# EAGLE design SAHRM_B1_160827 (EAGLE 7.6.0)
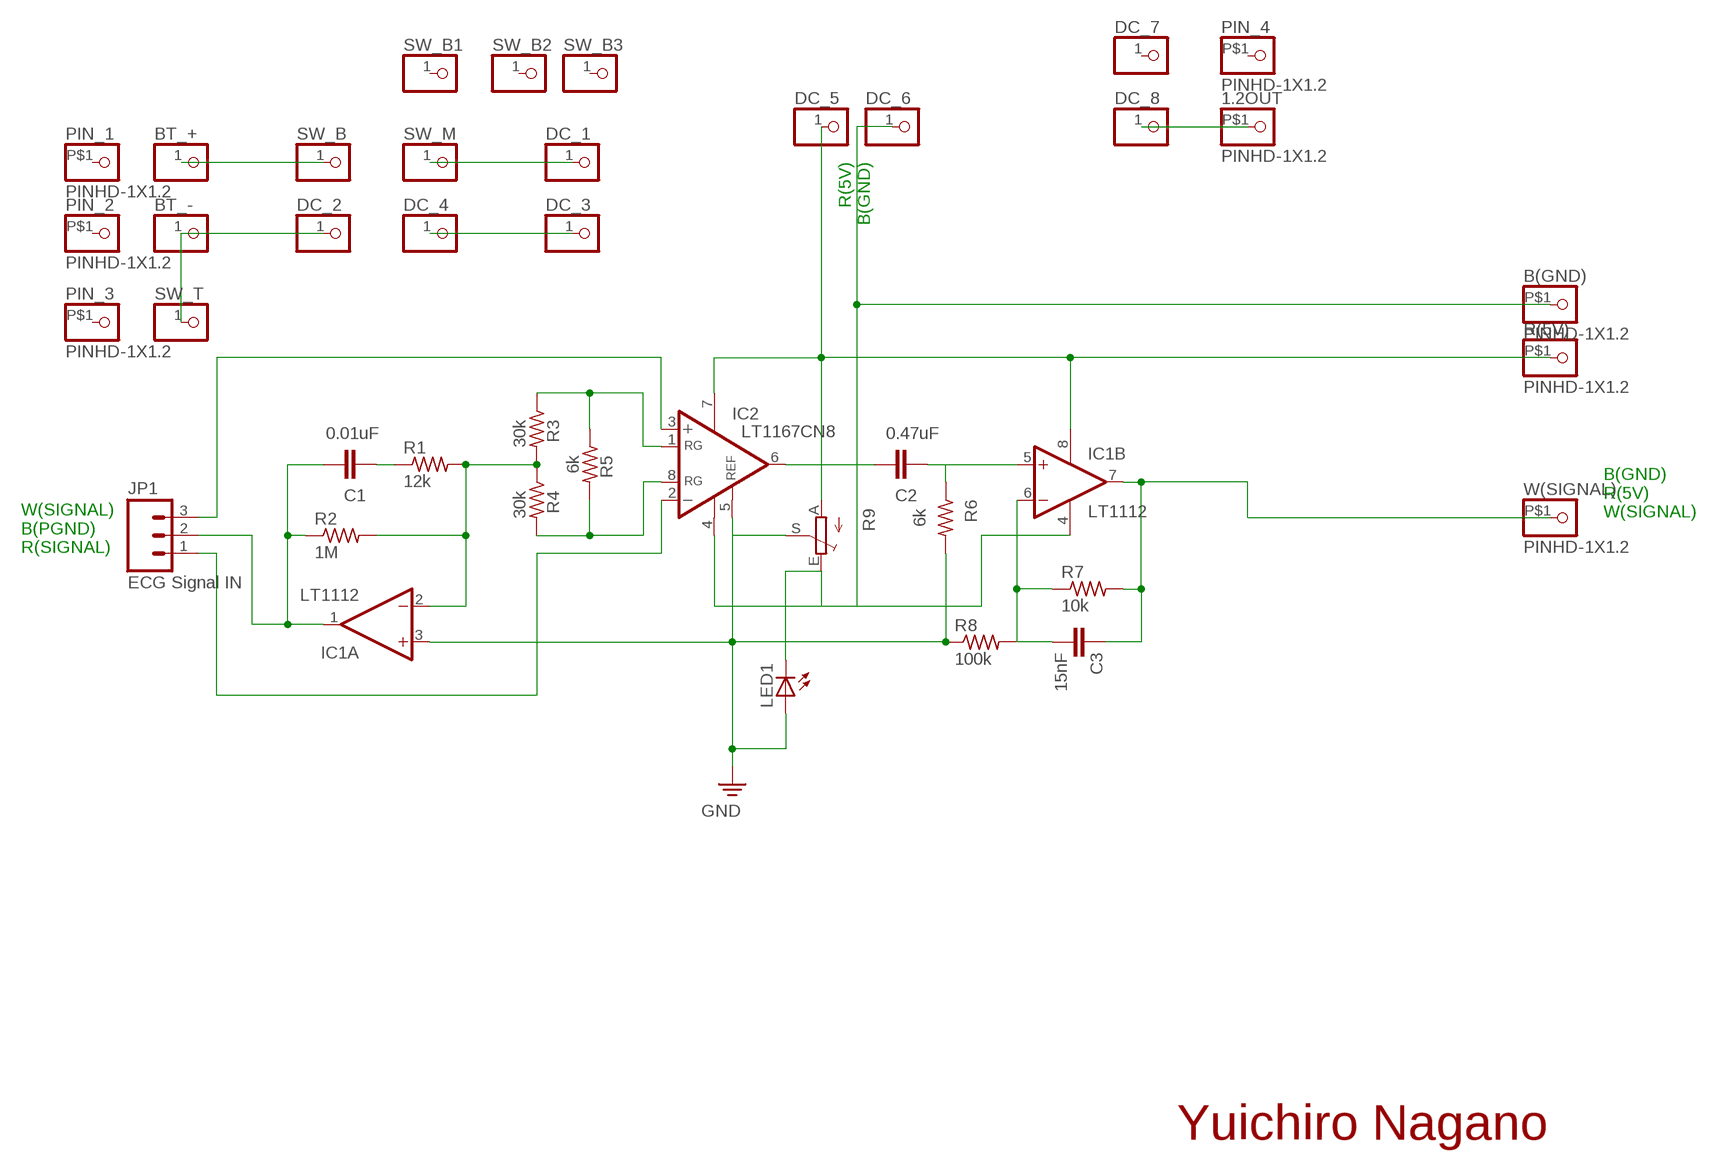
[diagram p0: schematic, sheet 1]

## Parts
1.2OUT  PINHD-1X1.2  [1X01.2]
B(GND)  PINHD-1X1.2  [1X01.2]
BT_+  PINHD-1X1  [1X01]
BT_-  PINHD-1X1  [1X01]
C1  0.01uF  C2,5-3  [C2.5-3]
C2  0.47uF  C2,5-3  [C2.5-3]
C3  15nF  C2,5-3  [C2.5-3]
DC_1  PINHD-1X1  [1X01]
DC_2  PINHD-1X1  [1X01]
DC_3  PINHD-1X1  [1X01]
DC_4  PINHD-1X1  [1X01]
DC_5  PINHD-1X1  [1X01]
DC_6  PINHD-1X1  [1X01]
DC_7  PINHD-1X1  [1X01]
DC_8  PINHD-1X1  [1X01]
IC1  LT1112  2AMP_P8+4N  [DIL08]
IC2  LT1167CN8  LT1168CN8  [DIL08]
JP1  ECG Signal IN  M03PTH  [1X03]
LED1  LED3MM  [LED3MM]
PIN_1  PINHD-1X1.2  [1X01.2]
PIN_2  PINHD-1X1.2  [1X01.2]
PIN_3  PINHD-1X1.2  [1X01.2]
PIN_4  PINHD-1X1.2  [1X01.2]
R1  12k  R-US_0204/2V  [0204V]
R2  1M  R-US_0204/2V  [0204V]
R3  30k  R-US_0204/2V  [0204V]
R4  30k  R-US_0204/2V  [0204V]
R5  6k  R-US_0204/2V  [0204V]
R6  6k  R-US_0204/2V  [0204V]
R7  10k  R-US_0204/2V  [0204V]
R8  100k  R-US_0204/2V  [0204V]
R9  TRIM_EU-B25P  [B25P]
R(5V)  PINHD-1X1.2  [1X01.2]
SW_B  PINHD-1X1  [1X01]
SW_B1  PINHD-1X1  [1X01]
SW_B2  PINHD-1X1  [1X01]
SW_B3  PINHD-1X1  [1X01]
SW_M  PINHD-1X1  [1X01]
SW_T  PINHD-1X1  [1X01]
W(SIGNAL)  PINHD-1X1.2  [1X01.2]

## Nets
B1: IC1.3(A:+IN) IC2.5(REF) LED1.A R6.2 R8.1 R9.S ; supply symbol labelled GND
N$1: C1.2 IC1.1(A:OUT) JP1.2 R2.1
N$2: IC2.3(+IN) JP1.3
N$3: IC1.2(A:-IN) R1.2 R2.2 R3.2 R4.1
N$4: IC2.1(RG) R3.1 R5.1
N$5: IC2.8(RG) R4.2 R5.2
N$6: IC2.2(-IN) JP1.1
N$7: 1.2OUT.P$1(1.1) DC_8.1
N$8: C2.2 IC2.6(OUT)
N$9: C2.1 IC1.5(B:+IN) R6.1
N$10: C3.2 IC1.6(B:-IN) R7.1 R8.2
N$11: C1.1 R1.1
N$15: DC_5.1 IC1.8(P:V+) IC2.7(V+) R9.A R(5V).P$1(1.1)
N$16: C3.1 IC1.7(B:OUT) R7.2 W(SIGNAL).P$1(1.1)
N$17: B(GND).P$1(1.1) DC_6.1 IC1.4(P:V-) IC2.4(V-) LED1.K(C) R9.E
N$27: BT_+.1 SW_B.1
N$28: BT_-.1 DC_2.1 SW_T.1
N$34: DC_1.1 SW_M.1
N$37: DC_3.1 DC_4.1
Unconnected: DC_7.1 PIN_1.P$1(1.1) PIN_2.P$1(1.1) PIN_3.P$1(1.1) PIN_4.P$1(1.1) SW_B1.1 SW_B2.1 SW_B3.1

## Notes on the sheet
- R(5V)
  B(GND)
- B(GND)
  R(5V)
  W(SIGNAL)
- W(SIGNAL)
  B(PGND)
  R(SIGNAL)
- Yuichiro Nagano

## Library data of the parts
1.2OUT B(GND) PIN_1-PIN_4 R(5V) W(SIGNAL) = pinhead:PINHD-1X1.2
BT_+ BT_- DC_1-DC_8 SW_B SW_B1-SW_B3 SW_M SW_T = adafruit:PINHD-1X1: Pin header 1x1 for 0.1" spacing
C1-C3 = capacitor-wima:C: CAPACITOR
IC1 = linear:2AMP_P8+4: OP AMP
IC2 = linear-technology:LT1168: Low Power, Single Resistor Gain Programmable, Precision Instrumentation Amplifier SourcE: LT1168.pdf; MPN: LT1168CN8#PBF; OC_FARNELL: 1330587; OC_NEWARK: 57M2327
JP1 = SparkFun-Connectors:M03: Header 3 Standard 3-pin 0.1" header. Use with straight break away headers (SKU : PRT-00116), right angle break away headers (PRT-00553), swiss pins (PRT-00743), machine pins (PRT-00117), and female headers (PRT-00115). Molex polarized connector foot print use with SKU : PRT-08232 with associated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
LED1 = adafruit:LED: LED
R1-R8 = resistor:R-US_: RESISTOR, American symbol
R9 = pot:TRIM_EU-: POTENTIOMETER

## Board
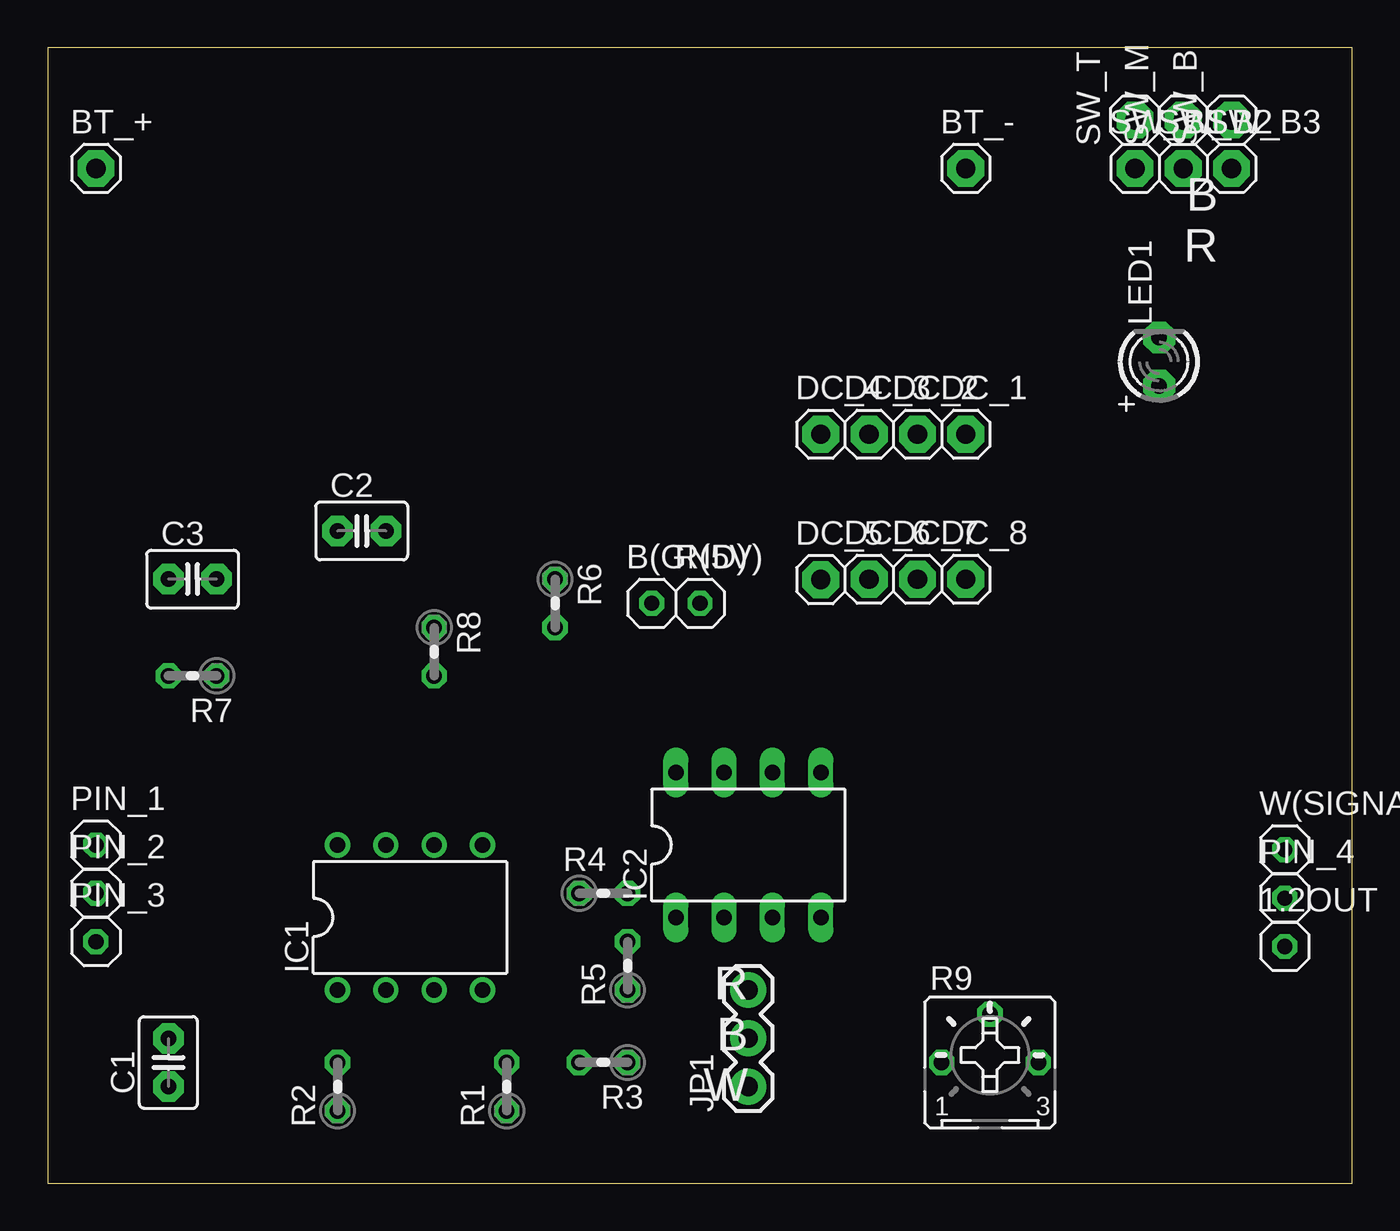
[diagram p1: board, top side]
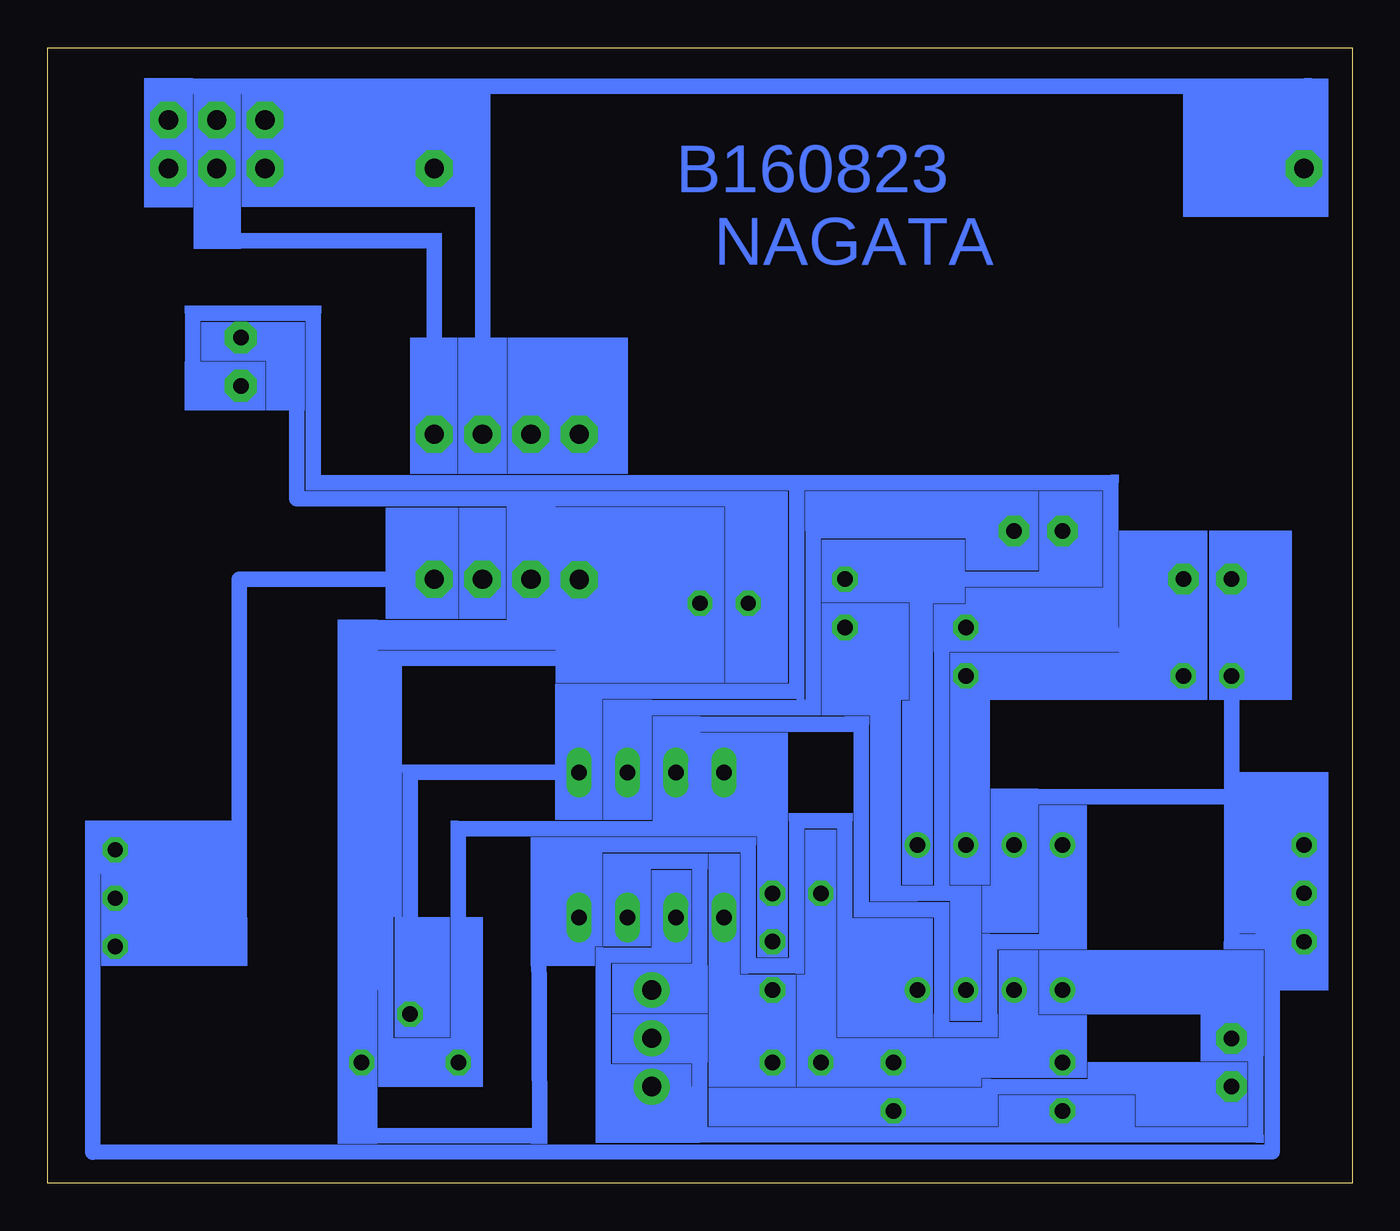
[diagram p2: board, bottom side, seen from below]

Size 68.58 x 59.69 mm. Coordinates in mm from the lower left corner, seen from the top.
Outline: 0,0 68.58,0 68.58,59.69 0,59.69 0,0
Copper layers (1*16): Top 0.035mm / dielectric 1.5mm / Bottom 0.035mm
Design rules "Fusion_eagle_rule_v1.1 *": minimum track width 32mil, minimum drill 12mil, track to track 6mil, track to pad 6mil, pad to pad 6mil, via to via 6mil, smd to smd 0mil, copper to edge 10mil, drill to drill 10mil, minimum pad ring 10mil, minimum via ring 6mil, stop-mask expansion 2mil, vias tented up to drill 100mil, thermal gap 10mil

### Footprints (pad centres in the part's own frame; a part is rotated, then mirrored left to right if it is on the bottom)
1X01.2 = drill 0.8 octagon: P$1 0,0
1X01 = drill 1.016 pad 1.93 octagon: 1 0,0
C2.5-3 = drill 0.813 pad 1.6 octagon: 1 -1.27,0; 2 1.27,0
DIL08 = drill 0.813 pad 1.27: 1 -3.81,-3.81; 2 -1.27,-3.81; 3 1.27,-3.81; 4 3.81,-3.81; 5 3.81,3.81; 6 1.27,3.81; 7 -1.27,3.81; 8 -3.81,3.81
DIL08' = drill 0.813 long: 1 -3.81,-3.81; 2 -1.27,-3.81; 3 1.27,-3.81; 4 3.81,-3.81; 5 3.81,3.81; 6 1.27,3.81; 7 -1.27,3.81; 8 -3.81,3.81
1X03 = drill 1.016 pad 1.88: 1 0,0; 2 2.54,0; 3 5.08,0
LED3MM = drill 0.813 pad 1.676 octagon: A -1.27,0; K 1.27,0
0204V = drill 0.813 octagon: 1 -1.27,0; 2 1.27,0
B25P = drill 0.813 octagon: A -2.54,0; E 2.54,0; S 0,2.54

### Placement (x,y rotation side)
1.2OUT  65.02,12.45 0 top
B(GND)  31.75,30.48 0 top
BT_+  2.54,53.34 0 top
BT_-  48.26,53.34 0 top
C1  6.35,6.35 90 top
C2  16.51,34.29 0 top
C3  7.62,31.75 0 top
DC_1  48.26,39.37 0 top
DC_2  45.72,39.37 0 top
DC_3  43.18,39.37 0 top
DC_4  40.64,39.37 0 top
DC_5  40.64,31.72 0 top
DC_6  43.18,31.75 0 top
DC_7  45.72,31.75 0 top
DC_8  48.26,31.75 0 top
IC1  19.05,13.97 0 top
IC2  LT1167CN8  [DIL08']  36.83,17.78 0 top
JP1  36.83,5.08 90 top
LED1  58.42,43.18 90 top
PIN_1  2.54,17.78 0 top
PIN_2  2.54,15.24 0 top
PIN_3  2.54,12.7 0 top
PIN_4  65.02,14.99 0 top
R1  24.13,5.08 90 top
R2  15.24,5.08 90 top
R3  29.21,6.35 180 top
R4  29.21,15.24 0 top
R5  30.48,11.43 90 top
R6  26.67,30.48 270 top
R7  7.62,26.67 180 top
R8  20.32,27.94 270 top
R9  49.53,6.35 0 top
R(5V)  34.29,30.48 0 top
SW_B  62.23,55.88 90 top
SW_B1  57.15,53.34 0 top
SW_B2  59.69,53.34 0 top
SW_B3  62.23,53.34 0 top
SW_M  59.69,55.88 90 top
SW_T  57.15,55.88 90 top
W(SIGNAL)  65.02,17.53 0 top

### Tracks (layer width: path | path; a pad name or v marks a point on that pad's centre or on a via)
B1
  Bottom 0.813: LED1.A 60.96,41.91 60.96,45.72 54.61,45.72 54.61,36.83 29.21,36.83 | 29.21,36.83 12.7,36.83 12.7,29.21 R8.1 21.59,29.21 21.59,15.24 | 29.21,36.83 29.21,25.86 40.64,25.86 IC2.5 49.53,21.59 R9.S | IC1.3 20.32,15.24 21.59,15.24 | R6.2 24.13,29.21 24.13,15.24 21.59,15.24
N$1
  Bottom 0.813: JP1.2 34.29,7.62 34.29,2.54 15.24,2.54 | 15.24,2.54 5.08,2.54 5.08,7.62 C1.2 6.35,10.16 IC1.1 | R2.1 15.24,2.54
N$2
  Bottom 0.813: IC2.3 38.1,16.92 34.29,16.92 34.29,10.16 JP1.3
N$3
  Bottom 0.813: 17.78,6.35 R1.2 R3.2 R4.1 | 17.78,6.35 R2.2 | 17.78,6.35 IC1.2
N$4
  Bottom 0.813: R3.1 R5.1 33.02,10.16 IC2.1
N$5
  Bottom 0.813: R5.2 R4.2 30.48,21.59 IC2.8
N$6
  Bottom 0.813: IC2.2 35.56,11.99 39.37,11.99 39.37,5.08 JP1.1
N$7
  Bottom 0.813: DC_8.1 58.5,31.75 58.5,12.42 65.02,12.42 1.2OUT.P$1
N$8
  Bottom 0.813: C2.2 28.35,34.29 28.35,24.99 38.1,24.99 IC2.6
N$9
  Bottom 0.813: C2.1 15.24,31.75 R6.1 22.86,31.75 IC1.5
N$10
  Bottom 0.813: C3.2 R7.1 R8.2 IC1.6
N$11
  Bottom 0.813: C1.1 19.05,5.08 19.05,3.81 R1.1
N$15
  Bottom 0.813: DC_5.1 40.64,30.48 | 40.64,30.48 40.64,27.58 50.8,27.58 50.8,6.35 R9.A 46.99,18.64 35.56,18.64 IC2.7 35.56,24.13 25.81,24.13 25.81,14.38 21.59,14.38 21.59,8.08 19.05,8.08 19.05,12.7 15.24,12.7 IC1.8 | R(5V).P$1 40.64,30.48
N$16
  Bottom 0.813: C3.1 R7.2 6.35,20.32 | 6.35,20.32 17.78,20.32 IC1.7 | 6.35,20.32 6.35,12.7 4.22,12.7 4.22,1.65 66.19,1.63 66.19,17.5 W(SIGNAL).P$1
N$17
  Bottom 0.813: 43.18,35.97 31.75,35.97 B(GND).P$1 | 43.18,35.97 DC_6.1 43.18,29.21 52.07,29.21 R9.E 52.02,2.49 42.72,2.49 42.77,13.97 IC2.4 40.64,17.78 31.75,17.78 31.75,11.43 29.21,11.43 29.21,19.05 26.67,19.05 26.67,10.16 IC1.4 | LED1.K 55.47,44.4 55.47,35.97 43.18,35.97
N$27
  Bottom 0.813: SW_B.1 62.23,57.66 2.54,57.66 BT_+.1
N$28
  Bottom 0.813: DC_2.1 45.72,53.34 BT_-.1 52.07,53.34 52.07,55.88 SW_T.1
N$34
  Bottom 0.813: SW_M.1 59.69,49.53 48.26,49.53 DC_1.1
N$37
  Bottom 0.813: DC_3.1 DC_4.1
(copper drawn outside any net)
  shapes: Bottom area x218

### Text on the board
Bottom: B160823 / NAGATA
tPlace: B / R | R / B / W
